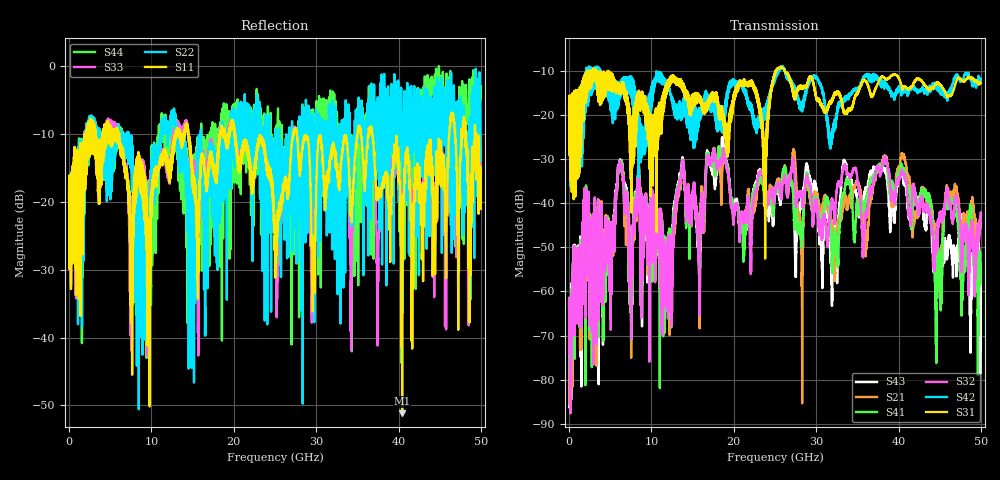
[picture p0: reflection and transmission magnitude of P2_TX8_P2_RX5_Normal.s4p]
!Keysight Technologies,N5225B,MY57041031,A.13.20.10
!Date: Friday, May 31, 2019 11:34:52
!Correction: S11(Full 4 Port(1,2,3,4))
!S12(Full 4 Port(1,2,3,4))
!S13(Full 4 Port(1,2,3,4))
!S14(Full 4 Port(1,2,3,4))
!S21(Full 4 Port(1,2,3,4))
!S22(Full 4 Port(1,2,3,4))
!S23(Full 4 Port(1,2,3,4))
!S24(Full 4 Port(1,2,3,4))
!S31(Full 4 Port(1,2,3,4))
!S32(Full 4 Port(1,2,3,4))
!S33(Full 4 Port(1,2,3,4))
!S34(Full 4 Port(1,2,3,4))
!S41(Full 4 Port(1,2,3,4))
!S42(Full 4 Port(1,2,3,4))
!S43(Full 4 Port(1,2,3,4))
!S44(Full 4 Port(1,2,3,4))
!S4P File: Measurements: <S11,S12,S13,S14>,
!<S21,S22,S23,S24>,
!<S31,S32,S33,S34>,
!<S41,S42,S43,S44>:
# Hz S  dB  R 50.0
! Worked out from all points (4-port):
!   5000 points, 10 MHz to 50 GHz, reference 50 ohm
!   strongest paths, dB at 10 MHz, 12.51 GHz, 25.01 GHz, 37.51 GHz, 50 GHz:
!     S31: -19.3, -11.7, -10.3, -12.8, -12.8
!     S42: -19.4, -17.0, -12.1, -11.5, -12.1
!     S32: -61.7, -53.9, -37.0, -31.8, -42.4
!     S41: -61.5, -56.0, -37.7, -32.3, -55.4
!     S21: -62.7, -56.5, -36.9, -32.0, -43.4
!     S43: -62.1, -52.8, -37.4, -32.0, -58.5
!   lowest |S11| = -51.2 dB at 40.44 GHz (marker M1), VSWR 1.01, Z = 50 - j0.272 ohm
!   |S11| at or under -10 dB: 20.17 GHz to 27.18 GHz (7.015 GHz wide, 29.6 % of centre); 27.67 GHz to 35.04 GHz (7.368 GHz wide, 23.5 % of centre); 36.81 GHz to 46.16 GHz (9.344 GHz wide, 22.5 % of centre)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
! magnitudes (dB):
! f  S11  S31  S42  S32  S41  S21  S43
! 10 MHz  -19.5  -19.3  -19.4  -61.7  -61.5  -62.7  -62.1
! 6.21 GHz  -11.9  -15.3  -12.5  -31.2  -30.8  -31.4  -30.6
! 11.62 GHz  -13.5  -14.4  -11.9  -62.2  -55.2  -62.0  -59.9
! 18.72 GHz  -10.1  -19.9  -22.0  -27.5  -27.8  -29.5  -25.6
! 31.86 GHz  -12.4  -17.3  -24.6  -39.9  -50.0  -44.6  -57.6
! 40.44 GHz  -51.2  -14.2  -14.8  -32.8  -31.7  -29.1  -33.2
! 50 GHz  -15.1  -12.8  -12.1  -42.4  -55.4  -43.4  -58.5
